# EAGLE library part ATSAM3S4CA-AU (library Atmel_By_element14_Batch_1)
AT91 ARM Cortex M3-based Processor
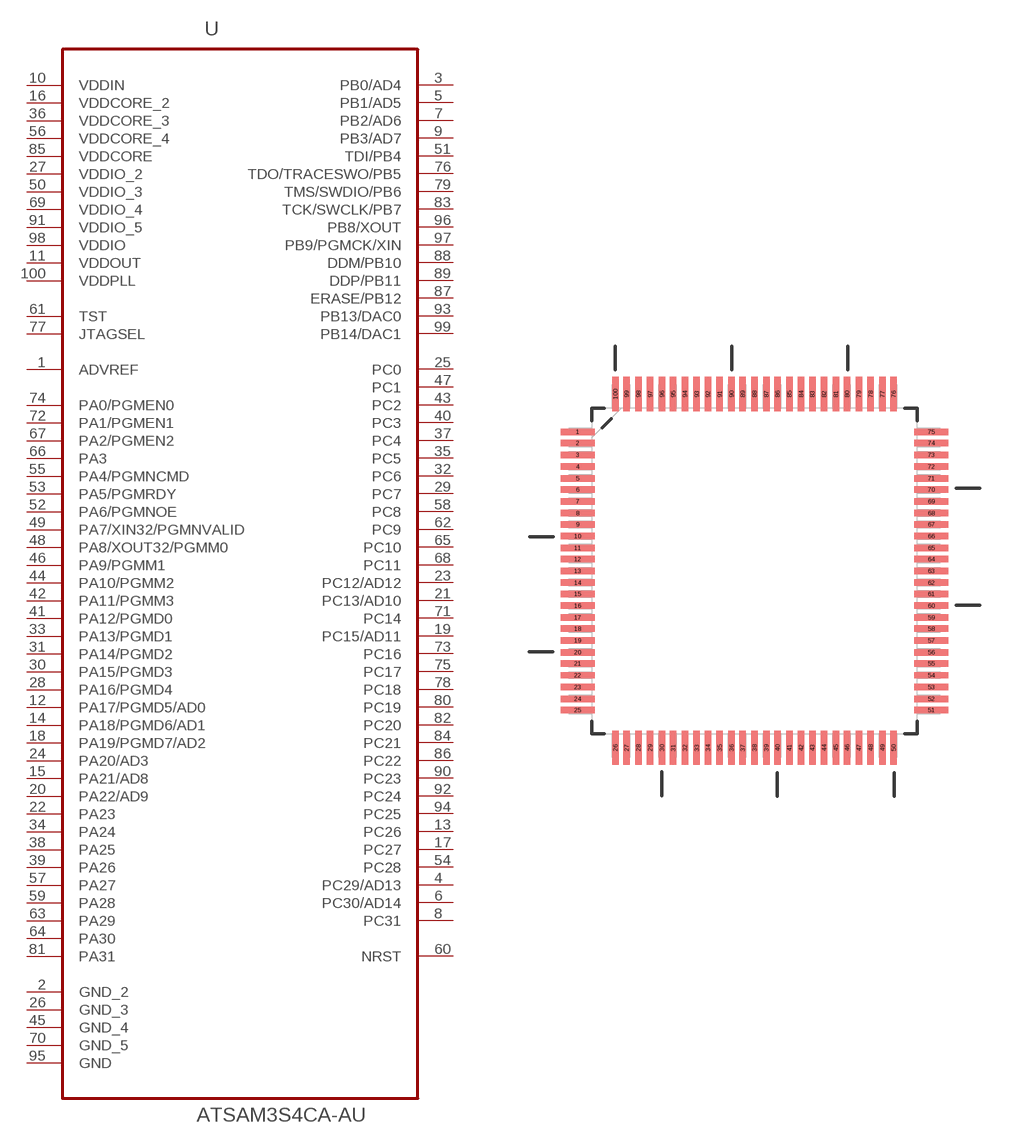
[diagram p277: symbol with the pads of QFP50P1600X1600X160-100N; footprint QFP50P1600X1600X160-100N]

Designator prefix U

## ATSAM3S4CA-AU (DESCRIPTION: AT91 ARM Cortex M3-based Processor; MPN: ATSAM3S4CA-AU; OC_FARNELL: 1841657; OC_NEWARK: 12T1315; PACKAGE: LQFP-100; SUPPLIER: Atmel Corporation)  [QFP50P1600X1600X160-100N]
1  ADVREF  pas
2  GND_2  pas
3  PB0/AD4
4  PC29/AD13
5  PB1/AD5
6  PC30/AD14
7  PB2/AD6
8  PC31
9  PB3/AD7
10  VDDIN  pwr
11  VDDOUT  pwr
12  PA17/PGMD5/AD0
13  PC26
14  PA18/PGMD6/AD1
15  PA21/AD8
16  VDDCORE_2  pwr
17  PC27
18  PA19/PGMD7/AD2
19  PC15/AD11
20  PA22/AD9
21  PC13/AD10
22  PA23
23  PC12/AD12
24  PA20/AD3
25  PC0
26  GND_3  pas
27  VDDIO_2  pwr
28  PA16/PGMD4
29  PC7
30  PA15/PGMD3
31  PA14/PGMD2
32  PC6
33  PA13/PGMD1
34  PA24
35  PC5
36  VDDCORE_3  pwr
37  PC4
38  PA25
39  PA26
40  PC3
41  PA12/PGMD0
42  PA11/PGMM3
43  PC2
44  PA10/PGMM2
45  GND_4  pas
46  PA9/PGMM1
47  PC1
48  PA8/XOUT32/PGMM0
49  PA7/XIN32/PGMNVALID
50  VDDIO_3  pwr
51  TDI/PB4
52  PA6/PGMNOE
53  PA5/PGMRDY
54  PC28
55  PA4/PGMNCMD
56  VDDCORE_4  pwr
57  PA27
58  PC8
59  PA28
60  NRST
61  TST  in
62  PC9
63  PA29
64  PA30
65  PC10
66  PA3
67  PA2/PGMEN2
68  PC11
69  VDDIO_4  pwr
70  GND_5  pas
71  PC14
72  PA1/PGMEN1
73  PC16
74  PA0/PGMEN0
75  PC17
76  TDO/TRACESWO/PB5
77  JTAGSEL  in
78  PC18
79  TMS/SWDIO/PB6
80  PC19
81  PA31
82  PC20
83  TCK/SWCLK/PB7
84  PC21
85  VDDCORE  pwr
86  PC22
87  ERASE/PB12
88  DDM/PB10
89  DDP/PB11
90  PC23
91  VDDIO_5  pwr
92  PC24
93  PB13/DAC0
94  PC25
95  GND  pas
96  PB8/XOUT
97  PB9/PGMCK/XIN
98  VDDIO  pwr
99  PB14/DAC1
100  VDDPLL  pwr

## Footprint QFP50P1600X1600X160-100N (pad centres in mm)
smd 1.473 x 0.279: 1 -7.62,5.994; 2 -7.62,5.512; 3 -7.62,5.004; 4 -7.62,4.496; 5 -7.62,3.988; 6 -7.62,3.505; 7 -7.62,2.997; 8 -7.62,2.489; 9 -7.62,2.007; 10 -7.62,1.499; 11 -7.62,0.991; 12 -7.62,0.508; 13 -7.62,0; 14 -7.62,-0.508; 15 -7.62,-0.991; 16 -7.62,-1.499; 17 -7.62,-2.007; 18 -7.62,-2.489; 19 -7.62,-2.997; 20 -7.62,-3.505; 21 -7.62,-3.988; 22 -7.62,-4.496; 23 -7.62,-5.004; 24 -7.62,-5.512; 25 -7.62,-5.994; 51 7.62,-5.994; 52 7.62,-5.512; 53 7.62,-5.004; 54 7.62,-4.496; 55 7.62,-3.988; 56 7.62,-3.505; 57 7.62,-2.997; 58 7.62,-2.489; 59 7.62,-2.007; 60 7.62,-1.499; 61 7.62,-0.991; 62 7.62,-0.508; 63 7.62,0; 64 7.62,0.508; 65 7.62,0.991; 66 7.62,1.499; 67 7.62,2.007; 68 7.62,2.489; 69 7.62,2.997; 70 7.62,3.505; 71 7.62,3.988; 72 7.62,4.496; 73 7.62,5.004; 74 7.62,5.512; 75 7.62,5.994
smd 0.279 x 1.473: 26 -5.994,-7.62; 27 -5.512,-7.62; 28 -5.004,-7.62; 29 -4.496,-7.62; 30 -3.988,-7.62; 31 -3.505,-7.62; 32 -2.997,-7.62; 33 -2.489,-7.62; 34 -2.007,-7.62; 35 -1.499,-7.62; 36 -0.991,-7.62; 37 -0.508,-7.62; 38 0,-7.62; 39 0.508,-7.62; 40 0.991,-7.62; 41 1.499,-7.62; 42 2.007,-7.62; 43 2.489,-7.62; 44 2.997,-7.62; 45 3.505,-7.62; 46 3.988,-7.62; 47 4.496,-7.62; 48 5.004,-7.62; 49 5.512,-7.62; 50 5.994,-7.62; 76 5.994,7.62; 77 5.512,7.62; 78 5.004,7.62; 79 4.496,7.62; 80 3.988,7.62; 81 3.505,7.62; 82 2.997,7.62; 83 2.489,7.62; 84 2.007,7.62; 85 1.499,7.62; 86 0.991,7.62; 87 0.508,7.62; 88 0,7.62; 89 -0.508,7.62; 90 -0.991,7.62; 91 -1.499,7.62; 92 -2.007,7.62; 93 -2.489,7.62; 94 -2.997,7.62; 95 -3.505,7.62; 96 -3.988,7.62; 97 -4.496,7.62; 98 -5.004,7.62; 99 -5.512,7.62; 100 -5.994,7.62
